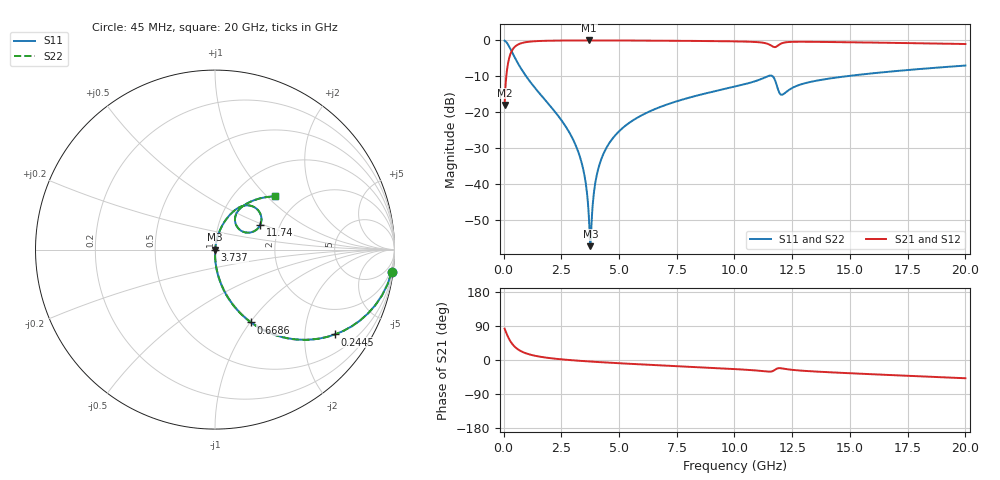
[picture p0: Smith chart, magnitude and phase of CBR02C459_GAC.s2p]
! S-parameter model data by Modelithics Inc.  support@modelithics.com 813-866-6335  Tampa FL USA
! S-Parameter data specifications:
! Substrate: 20-mil Rogers 4350B, substrate thickness, H=0.508mm, Dielectric constant, Er=3.75
! PCB Mounting Pad Footprint: Pad width, PadW=0.32mm , Pad length, PadL=0.37mm , Pad gap, PadG (edge-to-edge)=0.19mm , Reference planes=0.93mm apart
#  GHz  S  MA  R 50
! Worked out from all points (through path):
!   801 points, 45 MHz to 20 GHz, reference 50 ohm
!   highest |S21| = -0.01 dB at 3.712 GHz (marker M1); lowest = -17.9 dB at 45 MHz (marker M2)
!   group delay of S21, straight-line fit = 9.19 ps
!   lowest |S11| = -57.2 dB at 3.762 GHz (marker M3), VSWR 1.00, Z = 50.1 + j0.00391 ohm
!   |S11| at or under -10 dB: 981.5 MHz to 11.42 GHz (10.44 GHz wide, 168 % of centre); 11.66 GHz to 14.79 GHz (3.132 GHz wide, 23.7 % of centre)
!   |S22| runs from -57.2 to -0.1 dB; largest |S21 - S12| = 0
!   S11 on the Smith chart (normalised r, x): 45 MHz: 1, -16; 244.6 MHz: 0.99, -2.84; 668.6 MHz: 0.99, -1.01; 3.737 GHz: 1.00, -0.00; 11.74 GHz: 1.59, +0.47; 20 GHz: 1.51, +1.12
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0.045  0.9919 -7.3  0.1271 82.6  0.1271 82.6  0.9919 -7.3
0.24455  0.8193 -35.2  0.5728 54.8  0.5728 54.8  0.8193 -35.2
0.668594  0.4532 -63.7  0.8905 26.2  0.8905 26.2  0.4532 -63.7
1.292188  0.2331 -77.7  0.9714 12.1  0.9714 12.1  0.2331 -77.7
2.713981  0.06201 -88.2  0.9968 0.6  0.9968 0.6  0.06201 -88.2
3.387462  0.01961 -88.6  0.9984 -2.5  0.9984 -2.5  0.01961 -88.6
3.562069  0.0102 -85.6  0.9985 -3.3  0.9985 -3.3  0.0102 -85.6
3.711731  0.002743 -63.8  0.9986 -3.9  0.9986 -3.9  0.002743 -63.8
3.736675  0.001772 -42.9  0.9986 -4.0  0.9986 -4.0  0.001772 -42.9
3.761619  0.001387 1.6  0.9986 -4.1  0.9986 -4.1  0.001387 1.6
3.83645  0.004085 65.8  0.9985 -4.4  0.9985 -4.4  0.004085 65.8
4.060944  0.01463 79.3  0.9984 -5.2  0.9984 -5.2  0.01463 79.3
4.509931  0.03456 80.8  0.9979 -6.8  0.9979 -6.8  0.03456 80.8
5.358019  0.06845 79.0  0.996 -9.7  0.996 -9.7  0.06845 79.0
6.704981  0.1163 75.3  0.9914 -13.9  0.9914 -13.9  0.1163 75.3
10.0225  0.2285 65.1  0.9696 -24.0  0.9696 -24.0  0.2285 65.1
11.36946  0.3112 52.2  0.9096 -30.2  0.9096 -30.2  0.3112 52.2
11.74362  0.286 28.5  0.8065 -26.1  0.8065 -26.1  0.286 28.5
12.06789  0.1761 44.4  0.917 -22.3  0.917 -22.3  0.1761 44.4
13.36496  0.2684 58.6  0.956 -29.9  0.956 -29.9  0.2684 58.6
16.68248  0.3674 50.0  0.9265 -39.5  0.9265 -39.5  0.3674 50.0
20  0.4474 41.5  0.891 -48.2  0.891 -48.2  0.4474 41.5
